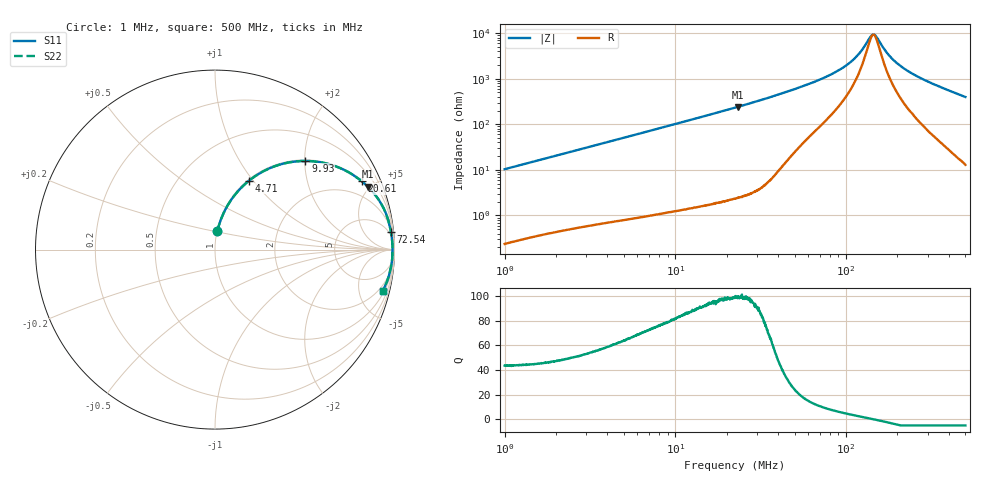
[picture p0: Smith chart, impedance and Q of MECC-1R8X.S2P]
!s-Parameter Generated by FASTRON Sdn. Bhd.
!FASTRON P/N : MECC-1R8X
!Keysight Technologies,E4991B,MY54100416,A.01.15
!Date: Mon Mar 16 14:48:26 2026
!Version  : Rev00 Mon Mar 16 14:48:26 2026
!Data & Calibration Information:
!PortZ  Port1:50+j0  Port2:50+j0
!When reading, reference impedance value at option line is always used.
!Remarks : This data is being provided solely for informational purposes.
!Freq	S11	S21	S12	S22
# Hz S dB R 50
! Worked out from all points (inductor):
!   1601 points, 1 MHz to 500 MHz, reference 50 ohm
!   read as one part in series: L = 1.64 uH near 1.032 MHz
!   highest Q = 99.3 at 23.25 MHz (marker M1), where L = 1.65 uH
!   self-resonance near 144.7 MHz
!   S11 on the Smith chart (normalised r, x): 1 MHz: 1.00, +0.21; 4.71 MHz: 1.02, +0.96; 9.93 MHz: 1.02, +2.02; 20.61 MHz: 1.04, +4.25; 72.54 MHz: 3, +20; 500 MHz: 1.26, -7.94
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1000000  -19.76 82.8  -0.07 -5.9  -0.07 -5.9  -19.76 82.8
2820919  -11.20 72.9  -0.39 -16.0  -0.39 -16.0  -11.20 72.9
4710377  -7.35 63.7  -0.95 -25.4  -0.95 -25.4  -7.35 63.7
7957584  -4.10 50.6  -2.23 -38.6  -2.23 -38.6  -4.10 50.6
9929607  -3.03 44.4  -3.10 -44.9  -3.10 -44.9  -3.03 44.4
1.381385e7  -1.82 35.2  -4.79 -54.2  -4.79 -54.2  -1.82 35.2
2.060919e7  -0.90 25.1  -7.45 -64.3  -7.45 -64.3  -0.90 25.1
2.236068e7  -0.77 23.3  -8.07 -66.2  -8.07 -66.2  -0.77 23.3
2.324629e7  -0.72 22.4  -8.37 -67.0  -8.37 -67.0  -0.72 22.4
3.647782e7  -0.30 14.0  -12.34 -75.1  -12.34 -75.1  -0.30 14.0
6.307767e7  -0.14 6.9  -18.33 -78.8  -18.33 -78.8  -0.14 6.9
7.254416e7  -0.13 5.6  -20.19 -78.7  -20.19 -78.7  -0.13 5.6
9.08741e7  -0.11 3.6  -23.86 -77.0  -23.86 -77.0  -0.11 3.6
1.082302e8  -0.10 2.2  -27.89 -72.4  -27.89 -72.4  -0.10 2.2
1.206648e8  -0.10 1.4  -31.57 -64.9  -31.57 -64.9  -0.10 1.4
1.376999e8  -0.09 0.4  -38.04 -31.5  -38.04 -31.5  -0.09 0.4
1.431536e8  -0.09 0.1  -39.41 -7.6  -39.41 -7.6  -0.09 0.1
1.505676e8  -0.09 -0.3  -38.53 26.5  -38.53 26.5  -0.09 -0.3
1.77937e8  -0.09 -1.6  -30.48 68.1  -30.48 68.1  -0.09 -1.6
2.086543e8  -0.10 -2.9  -25.65 75.8  -25.65 75.8  -0.10 -2.9
2.573461e8  -0.12 -4.8  -21.41 78.5  -21.41 78.5  -0.12 -4.8
5e8  -0.33 -14.0  -12.32 74.1  -12.32 74.1  -0.33 -14.0
